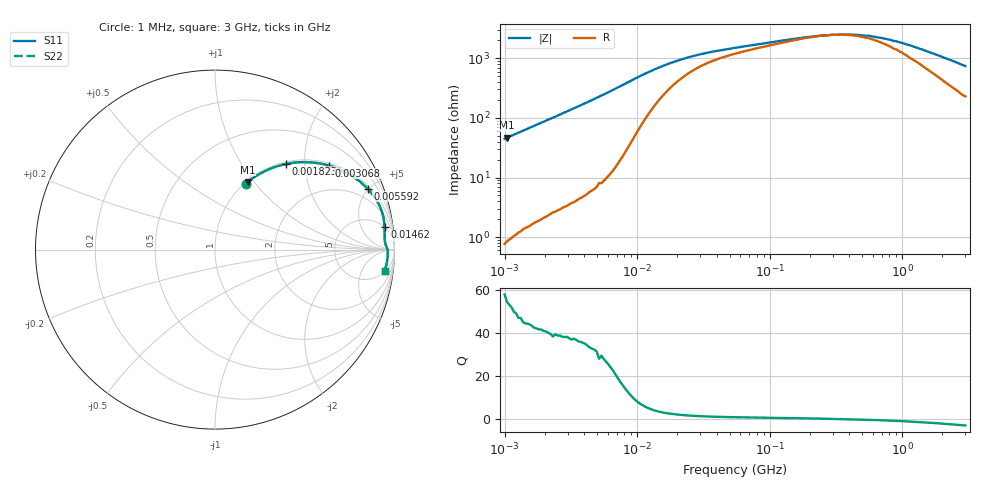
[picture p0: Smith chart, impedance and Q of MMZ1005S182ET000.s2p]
! S-parameter Generated by TDK Corporation
! Copyright(C) 2016 TDK Corporation.
! All Rights Reserved.
! TDK P/N: MMZ1005S182ET000 (Chip Beads)
! Property: |Z|=1800¶ at 100MHz
! Size(LxWxT): 1x0.5x0.5mm, 0.039x0.02x0.02inches
! Model Type: s2p (Touchstone File Format Version 1.0)
! Frequency: DC=Yes Start=1MHz Stop=3000MHz 202points Log-sweep
! Note: This model was converted from impedance.
! Model Generated on May. 16, 2016
! Hash(MD5):
! Port Assignments:
!  1 ---@@@--- 2
! Applicable Conditions:
!  Temperature = 25 degC
!  DC Bias Current = 0 A
!  Small Signal Operation
! Terms and conditions regarding TDK Simulation Models
! (1)This simulation model is being provided solely for informational purposes. Please refer to the specifications of the products in terms of detailed characteristics of such products.
! (2)In no event shall TDK Corporation of any of its subsidiaries be liable for any loss or damage arising, directly or indirectly,
!  From any information contained in this simulation model, including, but not limited to loss or damages arising from any inaccuracies, omissions or errors in connection with such information.
! (3)Any and all copyrights on this simulation model are owned by TDK Corporation.
!  Duplication or redistribution of this simulation model without prior written permission from TDK Corporation is prohibited.
! (4)This simulation model is subject to any modification or change without any prior notice.
! (5)Neither TDK Corporation nor any of its subsidiaries shall make any warranty, express or implied,
!  Including but not limited to the correctness, implied warranties of merchantability and fitness for a particular purpose with respect to this simulation models.
! (6)The use of this simulation model shall be deemed to have consented to the terms and conditions hereof.
# MHz S MA R 50
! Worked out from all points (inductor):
!   201 points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, 1 MHz to 3 GHz, reference 50 ohm
!   read as one part in series: L = 7.06 uH near 1.041 MHz
!   highest Q = 54.7 at 1.041 MHz (marker M1), where L = 7.11 uH
!   self-resonance near 296.1 MHz
!   S11 on the Smith chart (normalised r, x): 1 MHz: 1.02, +0.89; 1.823 MHz: 1.04, +1.60; 3.068 MHz: 1.07, +2.66; 5.592 MHz: 1.18, +4.93; 14.62 MHz: 5, +13; 3 GHz: 6, -14
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1  0.4051 65.1  0.9073 -23.9  0.9073 -23.9  0.4051 65.1
1.040844  0.4185 64.2  0.9006 -24.7  0.9006 -24.7  0.4185 64.2
1.377479  0.5156 57.7  0.8455 -31.0  0.8455 -31.0  0.5156 57.7
1.822989  0.6177 50.5  0.7717 -38.1  0.7717 -38.1  0.6177 50.5
2.412589  0.7155 42.9  0.6808 -45.7  0.6808 -45.7  0.7155 42.9
3.067588  0.7898 36.3  0.5928 -52.1  0.5928 -52.1  0.7898 36.3
3.900413  0.8508 30.1  0.502 -58.3  0.502 -58.3  0.8508 30.1
5.592179  0.9154 21.8  0.3711 -66.2  0.3711 -66.2  0.9154 21.8
6.83139  0.938 17.7  0.3048 -69.5  0.3048 -69.5  0.938 17.7
8.686058  0.9523 13.6  0.2354 -71.6  0.2354 -71.6  0.9523 13.6
14.61624  0.9526 7.5  0.1363 -65.9  0.1363 -65.9  0.9526 7.5
18.58443  0.9499 5.8  0.1106 -60.2  0.1106 -60.2  0.9499 5.8
25.59965  0.9477 4.2  0.08861 -51.8  0.08861 -51.8  0.9477 4.2
35.26298  0.9472 3.1  0.07508 -43.7  0.07508 -43.7  0.9472 3.1
54.77226  0.9487 2.2  0.06338 -34.9  0.06338 -34.9  0.9487 2.2
213.6344  0.9593 0.4  0.0413 -9.6  0.0413 -9.6  0.9593 0.4
294.2768  0.9612 0.0  0.03882 -0.2  0.03882 -0.2  0.9612 0.0
457.0858  0.9625 -0.6  0.03889 15.3  0.03889 15.3  0.9625 -0.6
558.3748  0.9633 -1.0  0.04018 23.4  0.04018 23.4  0.9633 -1.0
800.5644  0.9633 -1.7  0.04677 37.5  0.04677 37.5  0.9633 -1.7
1194.682  0.9625 -2.7  0.06015 50.1  0.06015 50.1  0.9625 -2.7
3000  0.9528 -7.0  0.1285 65.0  0.1285 65.0  0.9528 -7.0
